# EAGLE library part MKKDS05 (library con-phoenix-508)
PHOENIX
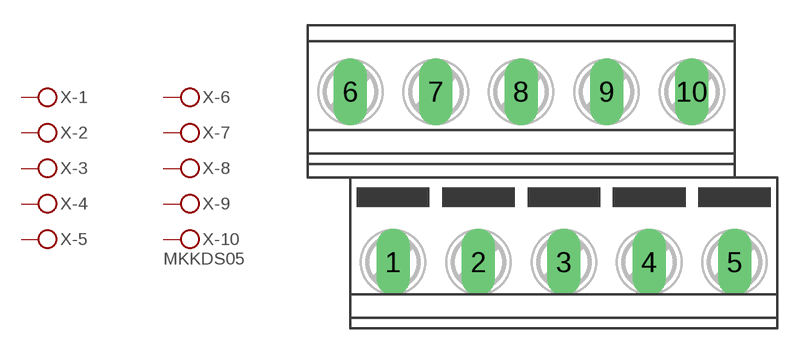
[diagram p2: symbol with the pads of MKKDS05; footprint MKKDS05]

Designator prefix X; gates -1=KL -2=KL -3=KL -4=KL -5=KL -6=KL -7=KL -8=KL -9=KL -10=KLV

## MKKDS05 (OC_FARNELL: unknown; OC_NEWARK: unknown)  [MKKDS05]
1  -1:KL  pas
2  -2:KL  pas
3  -3:KL  pas
4  -4:KL  pas
5  -5:KL  pas
6  -6:KL  pas
7  -7:KL  pas
8  -8:KL  pas
9  -9:KL  pas
10  -10:KL  pas

## Footprint MKKDS05 (pad centres in mm)
PHOENIX MKKDSN 1,5/ 8-5,08 Source: http://eshop.phoenixcontact.com .. 1726202.pdf
drill 1.321 long: 1 -8.89,-5.08; 2 -3.81,-5.08; 3 1.27,-5.08; 4 6.35,-5.08; 5 11.43,-5.08; 6 -11.43,5.08; 7 -6.35,5.08; 8 -1.27,5.08; 9 3.81,5.08; 10 8.89,5.08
